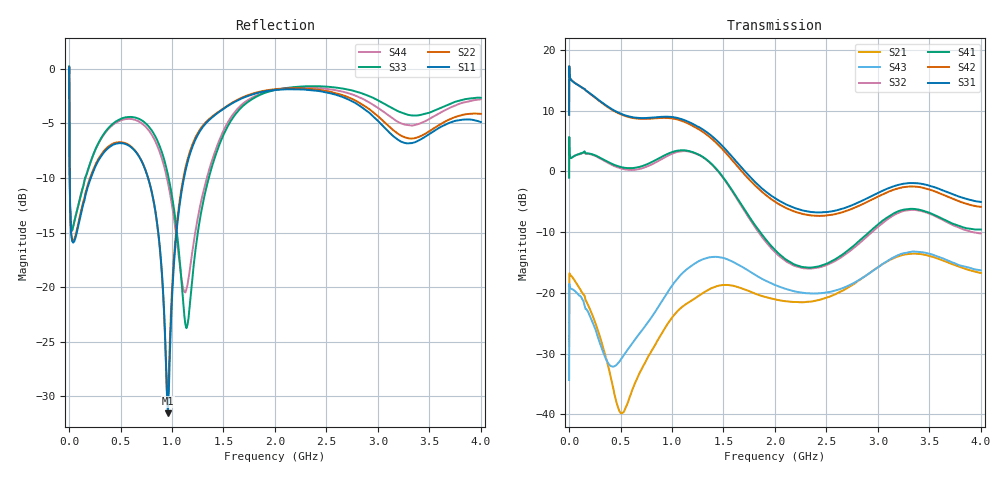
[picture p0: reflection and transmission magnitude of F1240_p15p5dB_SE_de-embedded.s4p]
! Integrated Device Technology
! Corporate Headquarters
! 6024 Silver Creek Valley Road
! San Jose, CA 95138  USA
! Phone:  1-408-284-8200
! Toll Free:  1-800-223-1366
! Webpage:  http://www.idt.com/
! Timing and RF Division
! 515 Groton Road, Suite 102
! Westford, MA 01886-6024
! Device:  F1240
! Description: Dual Intermediate Frequency Digital Variable Gain Amplifier
! Frequency:  10.0 -  500.00 MHz
! Package:  5x5 mm QFN Plastic Package: 32 pin
! Ports:  8 RF, 20 DC
!  Pin  1  = GA3 / Data  Pin 17  = RF OUT_B+
!  Pin  2  = GA4 / CLK  Pin 18  = RF OUT_B-
!  Pin  3  = GA5  Pin 19  = STBY_B
!  Pin  4  = VMODE  Pin 20  = Ground
!  Pin  5  = No Connect  Pin 21  = Ground
!  Pin  6  = GB5  Pin 22  = STB_A
!  Pin  7  = GB4  Pin 23  = RF OUT_A-  = Port 4
!  Pin  8  = GB3  Pin 24  = RF OUT_A+  = Port 3
!  Pin  9  = GB2  Pin 25  = GA0
!  Pin 10  = GB1  Pin 26  = ISET_A
!  Pin 11  = RF IN_B+  Pin 27  = VCC
!  Pin 12  = RF IN_B-  Pin 28  = Ground
!  Pin 13  = Ground  Pin 29  = RF IN_A-  = Port 2
!  Pin 14  = VCC  Pin 30  = RF IN_A+  = Port 1
!  Pin 15  = ISET_B  Pin 31  = GA1
!  Pin 16  = GB0  Pin 32  = GA2 / CSb
! Gain  = +19.5 dB
! State  = 1
! Voltage  = +5.00 V
! Current  = 85.292 mA (one channel only)
! Temperture  =  +25 C
! Test Date  =  2017-10-18
! Board  =  EB4031
! Data:  The device was measured on a custom evaluation board which has
!  individual transmission lines to the RF pins.  Data was collected
!  using a calibrated network analyzer.  The evaluation board was
!  de-embedded using Automatic Fixture Removal.
!  The reference plane is the edge of the package pin.
!  Only Channel A was measured.
!  This data is in single-ended operation.  If your needs are balanced
!  or differential S-parameters then this file needs to be used a
!  linear simulator.
! File Date:  2017-11-10  MJV
! Note:
!  Integrated Device Technology supplies this data as a sample of measured
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# Hz S dB R 100
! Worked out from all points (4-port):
!   410 points, 500 kHz to 4 GHz, reference 100 ohm
!   strongest paths, dB at 500 kHz, 930 MHz, 1.96 GHz, 2.98 GHz, 4 GHz:
!     S31: 9.3, 9.0, -4.0, -3.7, -5.0
!     S42: 9.3, 8.8, -4.5, -4.3, -5.8
!     S41: -1.0, 2.7, -12.2, -9.1, -9.6
!     S32: -1.0, 2.3, -12.6, -9.4, -10.2
!     S43: -34.4, -20.6, -18.4, -16.0, -16.3
!     S21: -28.8, -25.8, -20.9, -16.0, -16.7
!   lowest |S11| = -31.6 dB at 960 MHz (marker M1), VSWR 1.05, Z = 105 + j2.25 ohm
!   |S11| at or under -10 dB: 6.91 MHz to 211.4 MHz (204.4 MHz wide, 187 % of centre); 767.5 MHz to 1.116 GHz (348.9 MHz wide, 37 % of centre)
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500000  -0.32 -6.2  -28.73 8.0  -27.35 76.2  -61.39 64.6
        -28.81 7.7  -0.31 -6.2  -61.47 65.9  -27.35 77.3
        9.31 -105.3  -1.00 72.3  -0.42 1.0  -34.36 -157.4
        -1.01 73.4  9.29 -104.2  -34.36 -157.8  -0.43 3.3
3000000  -4.59 -55.5  -16.93 17.1  -19.13 13.8  -39.18 57.6
         -16.92 17.1  -4.56 -55.6  -39.15 57.8  -19.13 14.0
         16.78 -172.8  3.93 -6.0  -4.20 -51.1  -18.57 35.7
         3.93 -5.9  16.77 -172.6  -18.53 35.6  -4.26 -50.8
2.1e8  -10.03 -118.1  -22.92 -103.1  -21.95 -53.3  -33.84 6.5
       -22.99 -102.0  -9.85 -119.7  -33.82 6.6  -21.97 -53.3
       12.77 106.7  2.81 -56.4  -8.52 -83.5  -23.59 -112.1
       2.89 -56.5  12.72 105.9  -24.12 -110.1  -8.52 -82.7
5.5e8  -6.90 -174.6  -37.78 69.3  -23.57 -109.2  -27.90 -60.2
       -38.87 56.2  -6.83 -175.9  -28.04 -58.8  -23.72 -109.5
       9.20 22.4  0.31 -134.6  -4.45 -152.4  -30.32 69.4
       0.57 -135.7  9.09 21.4  -29.83 45.0  -4.61 -152.0
9.6e8  -31.56 23.9  -23.32 -49.7  -20.95 167.0  -23.36 -157.1
       -25.03 -57.8  -30.01 11.8  -23.69 -152.4  -21.38 166.4
       9.00 -77.8  2.59 135.6  -9.69 144.6  -20.19 -32.2
       2.91 130.8  8.80 -79.6  -19.82 -53.0  -10.42 148.9
1.51e9  -3.60 -145.0  -18.51 160.5  -26.74 37.2  -25.37 71.5
        -18.70 165.4  -3.56 -145.4  -25.28 77.3  -27.97 35.4
        3.81 123.2  -1.40 -44.7  -5.85 -126.9  -14.36 153.9
        -1.29 -49.7  3.29 121.8  -14.31 147.0  -5.47 -130.4
4e9  -4.89 -156.7  -16.77 60.2  -21.58 -43.1  -19.66 -48.3
     -16.73 59.5  -4.13 -150.8  -22.04 -29.5  -25.05 -29.3
     -5.03 4.6  -10.22 -125.6  -2.66 -136.7  -15.25 89.8
     -9.56 -136.3  -5.84 13.7  -16.29 63.2  -2.80 -142.0
